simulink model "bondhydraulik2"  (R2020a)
settings: Solver=ode45  StartTime=0.0  StopTime=2  RelTol=1e-3  EnableMultiTasking=on
undefined symbols (not defined in the file or in its folder): Display, Int, libbondgraph
libraries: libbondgraph x7

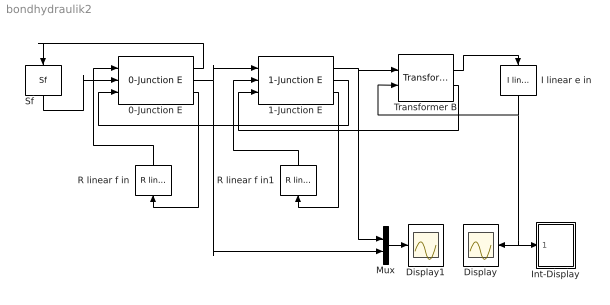
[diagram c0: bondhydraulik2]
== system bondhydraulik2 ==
  0-Junction E : libbondgraph/0-Junction E
  1-Junction E : libbondgraph/1-Junction E
  Display : Scope
  Display1 : Scope
  I linear e in : libbondgraph/I linear e in  I=500
  Int-Display : Subsystem  AncestorBlock=libbondgraph/Int-Display
  Mux : Mux  Inputs=2
  R linear f in : libbondgraph/R linear f in  R=1e9
  R linear f in1 : libbondgraph/R linear f in  R=8e7
  Sf : libbondgraph/Sf  f_ext=0.001
  Transformer B : libbondgraph/Transformer B  m=1000
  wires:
  Sf/1 -> 0-Junction E/2
  0-Junction E/1 -> Sf/1
  0-Junction E/3 -> R linear f in/1
  R linear f in/1 -> 0-Junction E/1
  0-Junction E/2 -> 1-Junction E/1, Mux/2
  1-Junction E/2 -> 0-Junction E/3
  Transformer B/1 -> I linear e in/1
  I linear e in/1 -> Transformer B/2, Display/1, Int-Display/1(In1)
  Mux/1 -> Display1/1
  1-Junction E/3 -> R linear f in1/1
  R linear f in1/1 -> 1-Junction E/2
  1-Junction E/1 -> Transformer B/1, Mux/1
  Transformer B/2 -> 1-Junction E/3

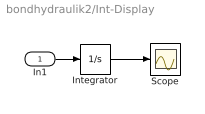
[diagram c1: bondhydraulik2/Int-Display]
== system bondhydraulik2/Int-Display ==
  In1 : Inport
  Integrator : Integrator
  Scope : Scope
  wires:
  Integrator/1 -> Scope/1
  In1/1 -> Integrator/1
